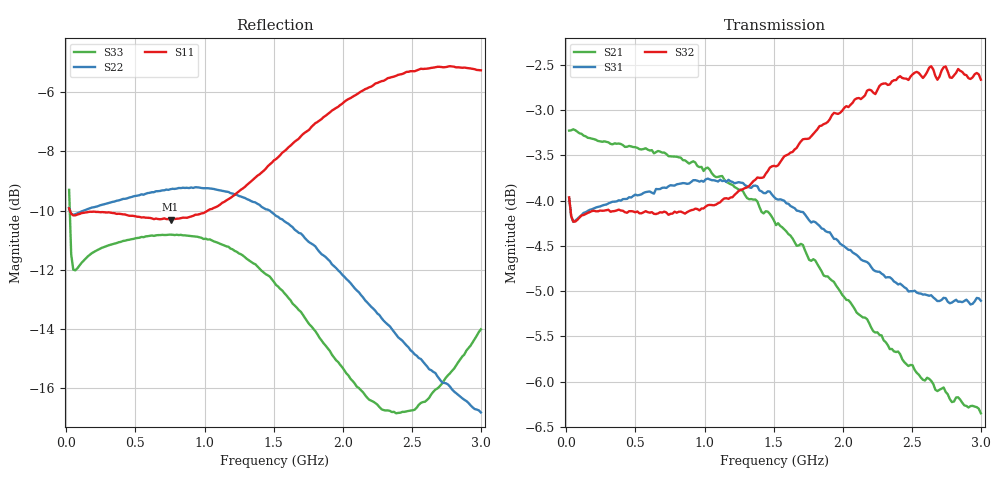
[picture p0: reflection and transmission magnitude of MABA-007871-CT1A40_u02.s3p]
#	MHz	S	RI	R	50
!FREQ	R1	I1	R2	I2	R3	I3
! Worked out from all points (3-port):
!   200 points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, 19.98 MHz to 3 GHz, reference 50 ohm
!   strongest paths, dB at 19.98 MHz, 768.7 MHz, 1.517 GHz, 2.266 GHz, 3 GHz:
!     S32: -4.0, -4.1, -3.6, -2.7, -2.7
!     S31: -4.0, -3.8, -4.0, -4.8, -5.1
!     S21: -3.2, -3.5, -4.3, -5.5, -6.4
!   lowest |S11| = -10.3 dB at 753.8 MHz (marker M1), VSWR 1.88, Z = 42.5 - j28.6 ohm
!   |S11| at or under -10 dB: 26.01 MHz to 1.024 GHz (997.7 MHz wide, 190 % of centre)
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19.975  0.3156 0.046  0.6858 -0.0724  -0.6256 -0.0991
        0.6859 -0.0733  0.3144 0.0574  0.6233 0.1103
        -0.6256 -0.0991  0.624 0.1096  0.255 0.229
49.925  0.3102 -0.00752  0.6882 -0.0598  -0.6141 -0.00629
        0.6884 -0.0594  0.3104 0.0193  0.6136 0.033
        -0.6141 -0.00629  0.6133 0.0335  0.2365 0.0853
94.85  0.3094 -0.0405  0.6819 -0.0864  -0.6169 0.0376
       0.6821 -0.0858  0.3138 0.0103  0.6174 0.0139
       -0.6169 0.0376  0.6173 0.0142  0.2485 0.0591
753.75  0.0136 -0.305  0.4481 -0.5007  -0.4253 0.4829
        0.4488 -0.4941  0.3347 -0.0776  0.6148 -0.0957
        -0.4253 0.4829  0.6129 -0.0962  0.2854 -0.0386
1128.125  -0.2412 -0.2191  0.1813 -0.6242  -0.1808 0.621
          0.1933 -0.6217  0.3072 -0.1492  0.6173 -0.1398
          -0.1808 0.621  0.6158 -0.1395  0.263 -0.0873
1517.475  -0.3831 0.0482  -0.1193 -0.5938  0.0982 0.6247
          -0.1045 -0.6026  0.2346 -0.2023  0.6318 -0.1993
          0.0982 0.6247  0.6277 -0.2007  0.2079 -0.1135
1876.875  -0.3179 0.3283  -0.3327 -0.4464  0.3044 0.525
          -0.3292 -0.469  0.1583 -0.2113  0.642 -0.2845
          0.3044 0.525  0.6372 -0.2803  0.1582 -0.0999
2281.2  -0.0635 0.5187  -0.455 -0.2172  0.4471 0.3615
        -0.4784 -0.2315  0.0929 -0.1864  0.6181 -0.4069
        0.4471 0.3615  0.6139 -0.3984  0.1347 -0.0569
2640.6  0.2043 0.5108  -0.4761 -0.00757  0.5175 0.2124
        -0.5016 -0.000275  0.0613 -0.1587  0.5502 -0.5166
        0.5175 0.2124  0.55 -0.508  0.1536 -0.0201
3000  0.4099 0.3594  -0.4271 0.1862  0.5517 0.0644
      -0.4337 0.2087  0.0425 -0.138  0.4432 -0.6033
      0.5517 0.0644  0.4451 -0.5861  0.1992 -0.00722
